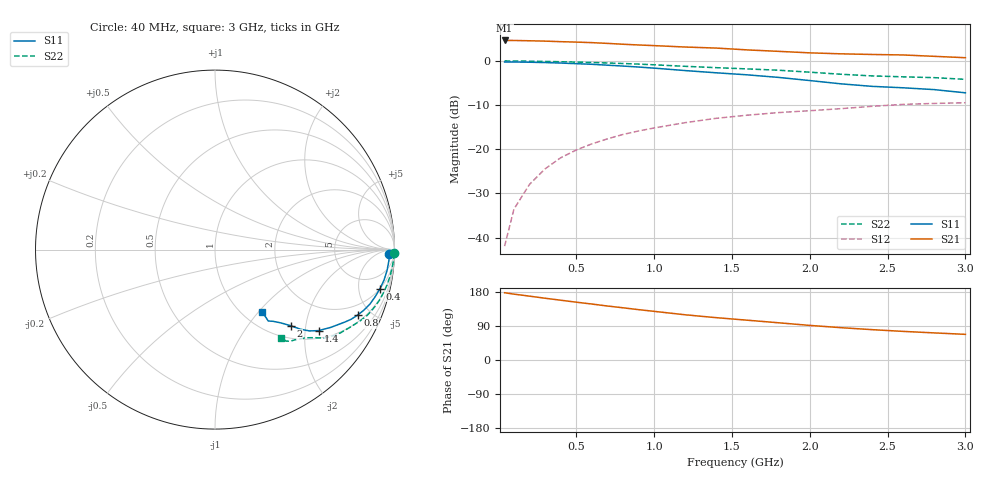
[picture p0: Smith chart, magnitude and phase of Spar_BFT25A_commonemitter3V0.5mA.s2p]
! Filename:  BFT25AH.S2P  Version:  2.0
! NXP part #: BFT25A  Date: Aug 1990
! Bias condition: Vce=3V, Ic=0.5mA
#  MHz  S  MA  R  50
! Freq  S11  S21  S12  S22  !GUM [dB]
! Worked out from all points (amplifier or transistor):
!   21 points, 40 MHz to 3 GHz, reference 50 ohm
!   highest |S21| = 4.6 dB at 40 MHz (marker M1)
!   |S21| within 3 dB of that: start of sweep to 2.176 GHz
!   unconditionally stable (mu >= 1): 2.742 GHz to end of sweep
!   at 300 MHz: K = 0.16, MSG = 14.5 dB, |S12| = -24.4 dB
!   at 1 GHz: K = 0.48, MSG = 9.3 dB, |S12| = -15.2 dB
!   at 3 GHz: K = 1.07, MAG = 3.5 dB, |S12| = -9.5 dB
!   S11 on the Smith chart (normalised r, x): 40 MHz: 43, -34; 400 MHz: 1.99, -8.09; 800 MHz: 1.34, -4.15; 1.4 GHz: 1.21, -2.36; 2 GHz: 1.25, -1.65; 3 GHz: 1.22, -1.04
40  0.972 -1.3  1.703 177.5  0.008 86.7  0.999 -1.2
100  0.971 -3.5  1.702 173.8  0.021 86.1  0.997 -3.0
200  0.966 -6.8  1.689 168.5  0.04 84.7  0.992 -5.9
300  0.957 -10.2  1.674 163.0  0.06 82.0  0.986 -8.9
400  0.945 -13.3  1.65 157.8  0.08 80.2  0.978 -11.7
500  0.93 -16.4  1.632 152.6  0.098 77.7  0.969 -14.4
600  0.915 -19.4  1.609 147.7  0.115 75.7  0.959 -17.0
700  0.894 -22.3  1.578 142.5  0.131 74.0  0.947 -19.4
800  0.874 -24.7  1.543 137.8  0.147 71.8  0.934 -21.7
900  0.852 -27.1  1.514 132.9  0.161 69.8  0.92 -23.9
1000  0.828 -29.2  1.489 128.4  0.174 68.1  0.903 -25.9
1200  0.777 -33.9  1.435 119.3  0.2 64.4  0.868 -29.9
1400  0.733 -38.0  1.396 111.7  0.224 61.7  0.838 -33.7
1600  0.695 -40.7  1.331 105.0  0.243 59.3  0.811 -36.5
1800  0.65 -43.0  1.282 98.2  0.26 57.4  0.784 -39.0
2000  0.599 -45.1  1.233 91.3  0.273 54.6  0.745 -41.2
2200  0.55 -48.0  1.202 85.3  0.288 52.3  0.706 -44.1
2400  0.515 -50.9  1.182 80.1  0.306 50.3  0.676 -47.7
2600  0.496 -53.3  1.167 75.5  0.322 48.9  0.66 -50.7
2800  0.473 -53.1  1.126 71.5  0.33 48.0  0.646 -52.1
3000  0.435 -52.9  1.086 67.7  0.336 47.4  0.618 -53.2
